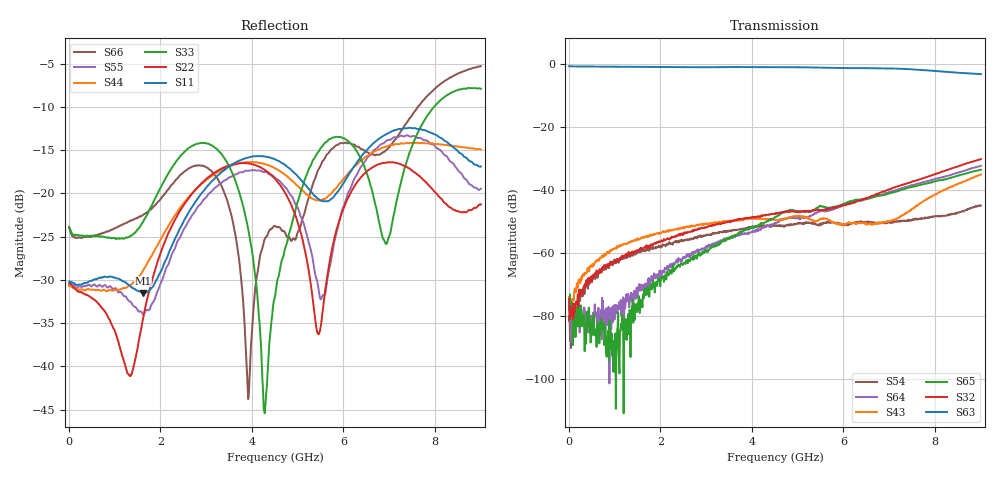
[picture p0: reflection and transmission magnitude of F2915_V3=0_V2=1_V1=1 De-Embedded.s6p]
! Integrated Device Technology
! Corporate Headquarters
! 6024 Silver Creek Valley Road
! San Jose, CA 95138  USA
! Phone:  1-408-284-8200
! Toll Free:  1-800-223-1366
! Webpage:  http://www.idt.com/
! Timing and RF Division
! 515 Groton Road, Suite 102
! Westford, MA 01886-6024
! Device:  F2915
! Description: High Reliability SP5T RF Switch
! Frequency:  0.05 -  8.GHz
! Package:  4x4 mm Thin QFN Plastic Package: 24 pin
! Ports:  6 RF,  5 DC
!  Pin  1  = GND
!  Pin  2  = RF5  =  Port 5
!  Pin  3  = GND
!  Pin  4  = GND
!  Pin  5  = RF4  =  Port 4
!  Pin  6  = GND
!  Pin  7  = GND
!  Pin  8  = RF3  =  Port 3
!  Pin  9  = GND
!  Pin 10  = GND
!  Pin 11  = RF2  =  Port 2
!  Pin 12  = GND
!  Pin 13  = GND
!  Pin 14  = RF1  =  Port 1
!  Pin 15  = GND
!  Pin 16  = Vcc
!  Pin 17  = V1
!  Pin 18  = V2
!  Pin 19  = V3
!  Pin 20  = VSSext
!  Pin 21  = GND
!  Pin 22  = RFC  =  Port 6
!  Pin 23  = GND
!  Pin 24  = GND
! Voltage:  VDD  =  +3.30 Volts
!  VSSEXT =  0.00 Volts
! Current:  IDD  = 275  uA
! State:  RF3 Selected
! V1:  Logic HIGH
! V2:  Logic HIGH
! V3:  Logic LOW
! Data:  The device was measured on the F291x evaluation board which has
!  individual transmission lines to the RF pins.  Data was collected
!  using a calibrated network analyzer.  The input lines were
!  modeled using Automatic Fixture Removal (AFR) from Keysight.
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# Hz S  dB  R 50
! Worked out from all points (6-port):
!   900 points, 10 MHz to 9 GHz, reference 50 ohm
!   strongest paths, dB at 10 MHz, 2.26 GHz, 4.51 GHz, 6.76 GHz, 9 GHz:
!     S63: -0.8, -1.1, -1.1, -1.4, -3.3
!     S32: -74.6, -55.2, -47.5, -41.2, -30.3
!     S65: -77.2, -65.2, -48.6, -42.0, -33.7
!     S43: -74.0, -52.9, -49.5, -50.6, -35.2
!     S64: -76.2, -63.6, -50.5, -41.8, -32.4
!     S54: -81.6, -57.0, -51.4, -50.6, -45.1
!   lowest |S11| = -31.5 dB at 1.62 GHz (marker M1), VSWR 1.05, Z = 49.5 + j2.6 ohm
!   |S11| at or under -10 dB: start of sweep to end of sweep
